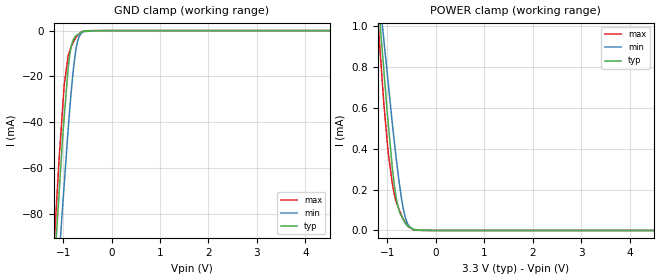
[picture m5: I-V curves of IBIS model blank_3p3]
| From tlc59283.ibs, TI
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|   blank_3p3 Model
[Model]   blank_3p3
Model_type   Input
Vinl = 0.99
Vinh = 2.31
|   typ   min   max
C_comp   5.648e-13   5.404e-13   5.892e-13
| Where nom  PVT is Nominal Process, 3.3V, 27C
|   Fast PVT is Strong Process,  3.6V, -40C
|   Slow PVT is Weak Process,   3V, 125C
[Voltage Range]   3.3   3   3.6
|Ambient Temperature   25   85   -40
|Junction Temperature
[Temperature Range]   27   125   -40
[Power Clamp Reference]   3.3   3   3.6
[GND Clamp Reference]   0   0   0
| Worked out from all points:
|   GND clamp passes 1 mA (typ) near -0.64 V on its own axis
|   POWER clamp passes 1 mA (typ) near -1.15 V on its own axis
[GND Clamp]
|   Voltage   I(typ)   I(min)   I(max)
-3.3V     -957.2mA   -926.2mA   -1.005A
-1.203V   -111.4mA   -138.9mA   -99.21mA
-1.168V   -98.74mA   -127.5mA   -86.49mA
-1.084V   -70.63mA   -99.76mA   -55.62mA
-1.032V   -53.53mA   -82.86mA   -39.88mA
-979.2mV  -37.86mA   -67.15mA   -23.78mA
-896.4mV  -16.09mA   -42.55mA   -10.8mA
-864.6mV  -10.47mA   -34.2mA    -8.856mA
-807mV    -4.883mA   -20.41mA   -5.678mA
-732mV    -2.18mA    -7.596mA   -2.824mA
-590.7mV  -305.7uA   -561.9uA   -382.9uA
6.6V      0A         0A         0A
[POWER Clamp]
|   Voltage   I(typ)   I(min)   I(max)
-3.3V     8.146mA    6.63mA     9.069mA
-1.213V   1.208mA    1.258mA    1.087mA
-1.142V   984.9uA    1.091mA    848.6uA
-1.076V   792.5uA    938.3uA    630.4uA
-986.4mV  532.1uA    728.1uA    386.6uA
-897.6mV  305.3uA    520.7uA    228.1uA
-821.7mV  164.8uA    360.7uA    142.5uA
-714mV    72.64uA    164.5uA    76.74uA
-627mV    33.96uA    60.96uA    38.39uA
-534mV    15.01uA    16.71uA    13.38uA
-453.6mV  2.741uA    5.423uA    1.489uA
6.6V      0A         0A         0A
